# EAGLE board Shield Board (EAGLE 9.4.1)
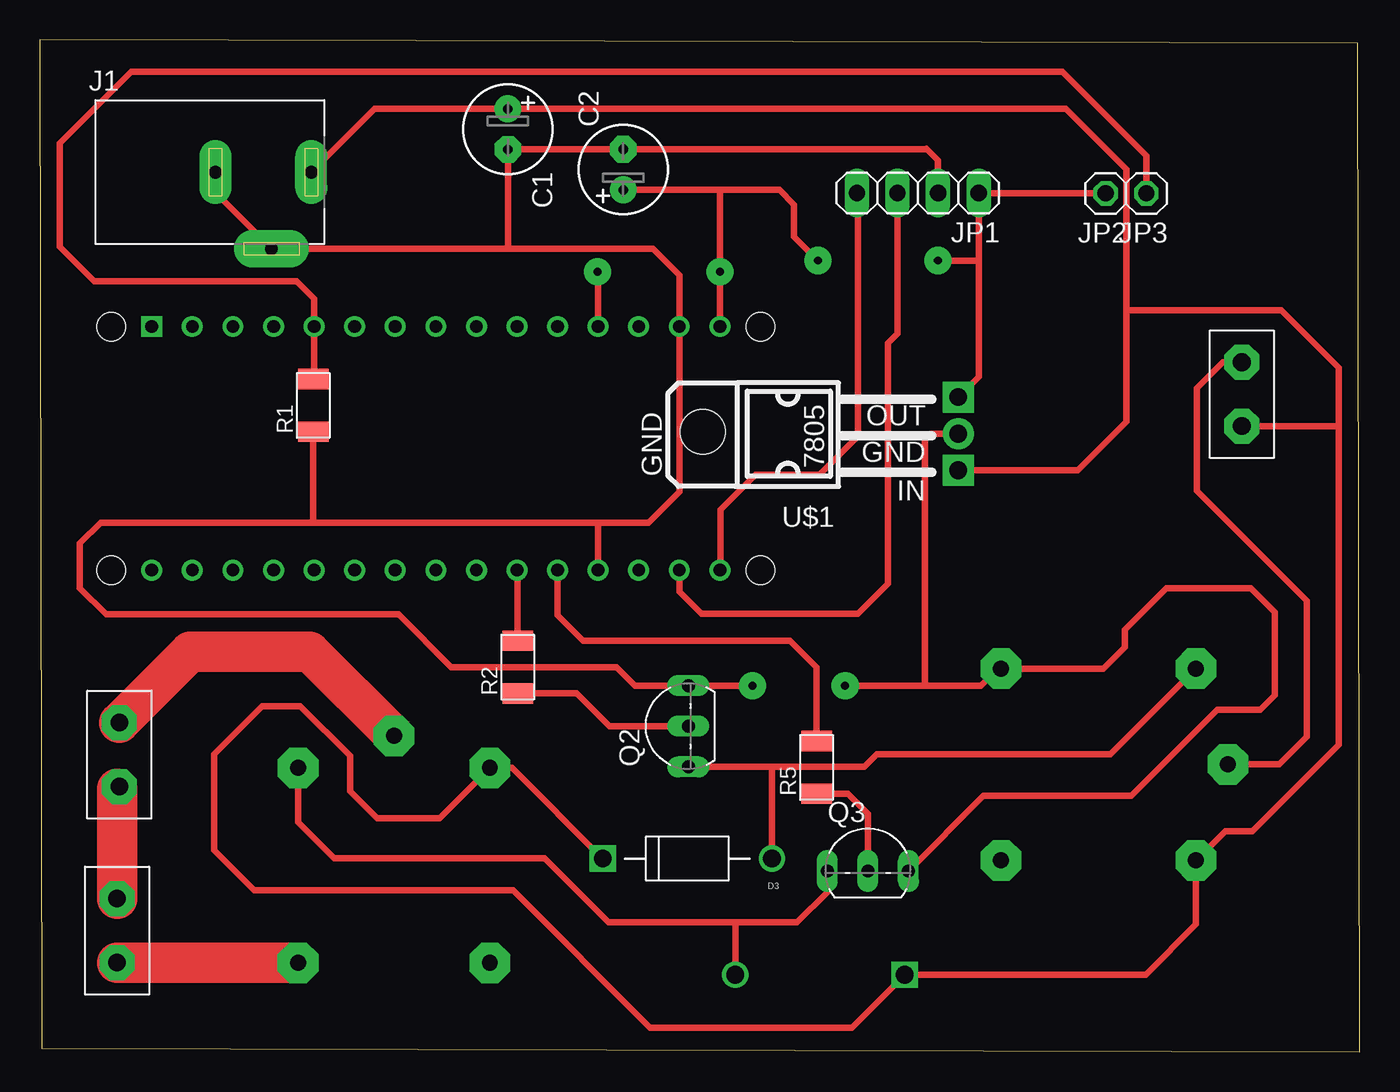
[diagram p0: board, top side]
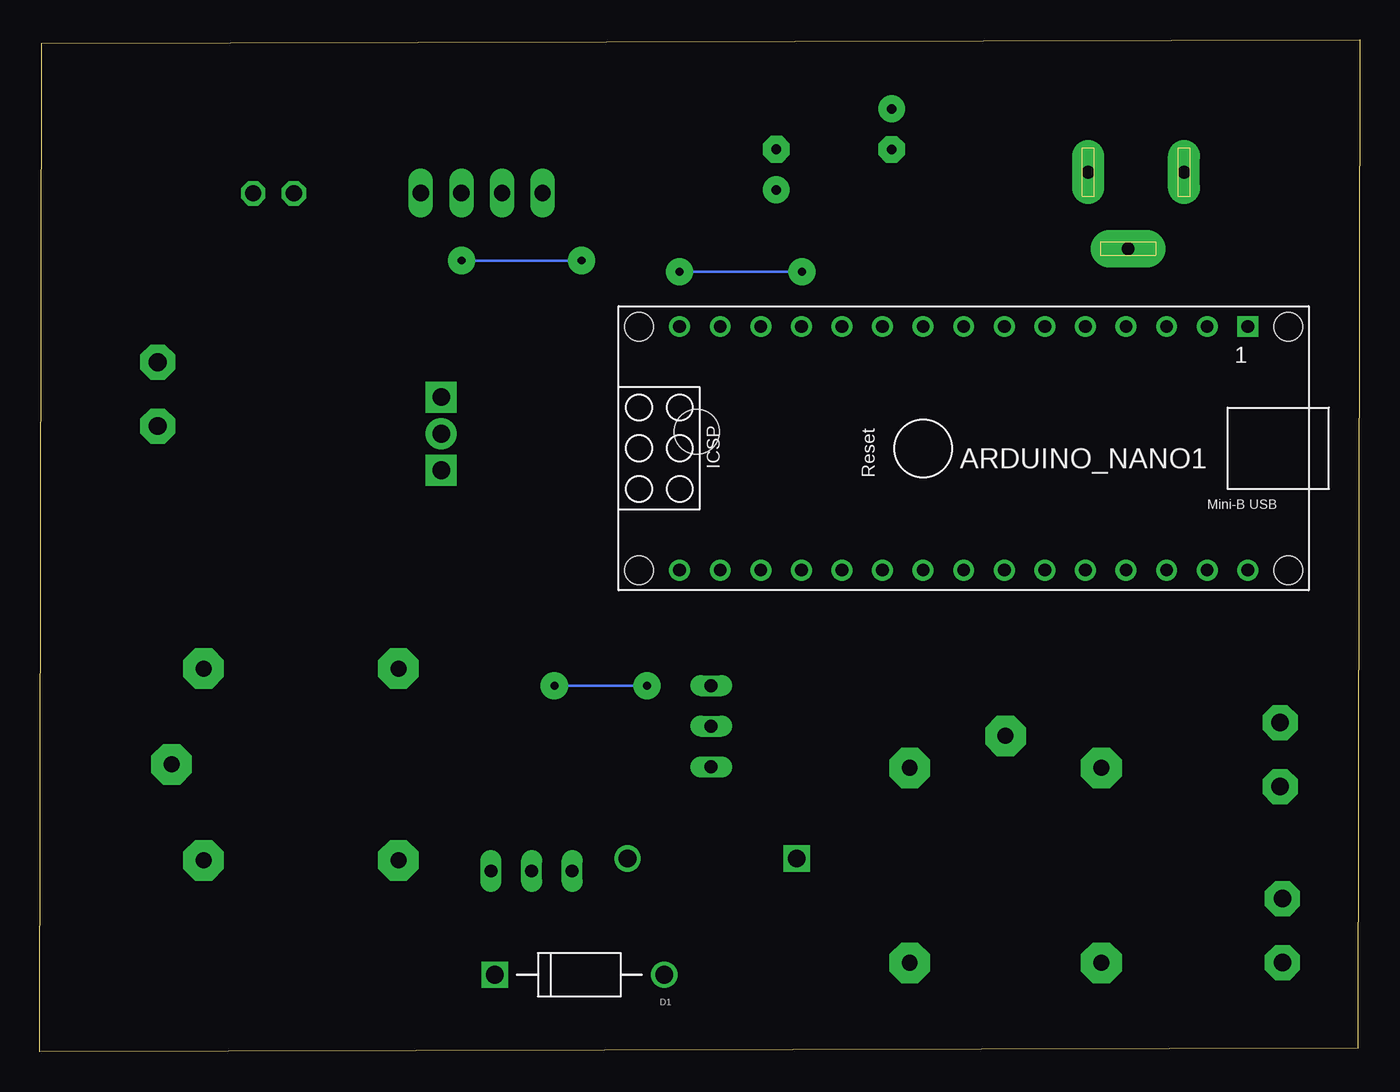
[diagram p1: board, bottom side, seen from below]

Size 82.6 x 63.3 mm. Coordinates in mm from the lower left corner, seen from the top.
Outline: 0.1,0.2 82.6,0 82.5,63.1 0,63.3 0.1,0.2
Copper layers (1*16): Top 0.035mm / dielectric 1.5mm / Bottom 0.035mm
Design rules "default": minimum track width 6mil, minimum drill 0.35mm, track to track 6mil, track to pad 6mil, pad to pad 6mil, via to via 6mil, smd to smd 6mil, copper to edge 40mil, drill to drill 6mil, minimum pad ring 10mil, minimum via ring 8mil, stop-mask expansion 4mil, vias tented up to drill 0mil, thermal gap 10mil

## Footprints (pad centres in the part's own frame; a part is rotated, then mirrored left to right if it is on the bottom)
ARDUINO_NANO = drill 0.8 square: 1 -20.32,-7.62 | drill 0.8: 2 -17.78,-7.62; 3 -15.24,-7.62; 4 -12.7,-7.62; 5 -10.16,-7.62; 6 -7.62,-7.62; 7 -5.08,-7.62; 8 -2.54,-7.62; 9 0,-7.62; 10 2.54,-7.62; 11 5.08,-7.62; 12 7.62,-7.62; 13 10.16,-7.62; 14 12.7,-7.62; 15 15.24,-7.62; 16 15.24,7.62; 17 12.7,7.62; 18 10.16,7.62; 19 7.62,7.62; 20 5.08,7.62; 21 2.54,7.62; 22 0,7.62; 23 -2.54,7.62; 24 -5.08,7.62; 25 -7.62,7.62; 26 -10.16,7.62; 27 -12.7,7.62; 28 -15.24,7.62; 29 -17.78,7.62; 30 -20.32,7.62 | hole 1.778: -22.86,-7.62; -22.86,7.62; 17.78,7.62; 17.78,-7.62
E2,5-6 = drill 0.6 pad 1.676: + -1.27,0 | drill 0.6 pad 1.676 octagon: - 1.27,0
DIOAD1060W80L520D270 = drill 1.1 pad 1.65: A 5.3,0 | drill 1.1 pad 1.65 square: C -5.3,0
NINIGI_DC-005 = drill 0.8 pad 2.35 long: 2 0,-4.8 | drill 0.8 pad 2 long: 3 -3.5,0; 4 2.5,0
1X04 = drill 1.016 long: 1 -3.81,0; 2 -1.27,0; 3 1.27,0; 4 3.81,0
1X01 = drill 1.016 octagon: 1 0,0
TO92-EBC = drill 0.813 long: B 0,-1.27; C -2.54,-1.27; E 2.54,-1.27
R1206FAB = smd 1.27 x 1.905: 1 -1.651,0; 2 1.651,0
L7805 = drill 1.1 pad 1.93: GND 0.127,-9.652 | drill 1.1 pad 1.93 square: IN -2.159,-9.652; OUT 2.413,-9.652 | hole 2.8: 0.254,6.35
RELAYSL = drill 1 pad 2.54 octagon: P$1 14.2,6; P$2 2,6; P$3 0,0; P$4 2,-6; P$5 14.2,-6
CNN = drill 1.1 pad 2.184 octagon: P$1 0,0; P$2 4,0

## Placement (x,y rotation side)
ARDUINO_NANO1  [ARDUINO_NANO]  27.32,37.75 180 bottom
C1  [E2,5-6]  29.29,57.72 270 top
C2  [E2,5-6]  36.51,55.19 90 top
D1  1N4007  [DIOAD1060W80L520D270]  48.83,4.81 0 bottom
D3  1N4007  [DIOAD1060W80L520D270]  40.52,12.08 0 top
J1  DC-005  [NINIGI_DC-005]  14.49,55.03 0 top
JP1  [1X04]  54.95,53.72 180 top
JP2  [1X01]  66.71,53.7 180 top
JP3  [1X01]  69.25,53.7 180 top
Q2  BC548  [TO92-EBC]  39.32,20.36 90 top
Q3  BC548  [TO92-EBC]  51.83,12.57 0 top
R1  1 K  [R1206FAB]  17.11,40.44 90 top
R2  1 K  [R1206FAB]  29.91,24.06 90 top
R5  1 K  [R1206FAB]  48.61,17.78 90 top
U$1  -L7805  [L7805]  47.83,38.54 90 top
U$3  RELAYSL  [RELAYSL]  74.36,17.97 180 top
U$5  RELAYSL  [RELAYSL]  22.16,19.75 270 top
U$6  CNN  [CNN]  4.83,9.57 270 top
U$7  CNN  [CNN]  4.97,16.58 90 top
U$8  CNN  [CNN]  75.23,43.14 270 top

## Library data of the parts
ARDUINO_NANO1 = ArduinoNanoV30
C1 C2 = Clean-Kong
D1 D3 = 1N4007; AVAILABILITY: Unavailable; DESCRIPTION: Diode, Standard Recovery, 1a, 1kv, Do-41, Full Reel; MF: Diodes; MP: 1N4007-T; PACKAGE: DO-41 Multicomp; PRICE: None
J1 = DC-005; AVAILABILITY: Unavailable; MF: Littelfuse Inc.; MP: DC-005; PACKAGE: 0603 Ninigi; PRICE: None
JP1-JP3 = pinhead
Q2 Q3 = transistor-npn
R1 R2 R5 = fab
U$1 = tango
U$3 U$5 = relay
U$6-U$8 = resistor-bourns

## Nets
5V: ARDUINO_NANO1.12 ARDUINO_NANO1.15 C2.+ JP1.1 JP2.1 U$1.OUT
GND: ARDUINO_NANO1.14 ARDUINO_NANO1.19 C1.- C2.- J1.2 J1.3 JP1.2 Q2.E Q3.E R1.1 U$1.GND U$3.P$5
N$3: D3.A Q2.C U$3.P$4
N$5: ARDUINO_NANO1.5 JP3.1 R1.2
N$6: Q2.B R2.1
N$8: ARDUINO_NANO1.21 R2.2
N$9: D1.A Q3.C U$5.P$4
N$11: Q3.B R5.1
N$12: ARDUINO_NANO1.20 R5.2
N$14: U$5.P$3 U$7.P$2
N$15: U$6.P$1 U$7.P$1
N$16: U$3.P$3 U$8.P$1
N$17: U$5.P$5 U$6.P$2
RX: ARDUINO_NANO1.16 JP1.4
TX: ARDUINO_NANO1.17 JP1.3
VCC: C1.+ D1.C D3.C J1.4 U$1.IN U$3.P$2 U$5.P$2 U$8.P$2

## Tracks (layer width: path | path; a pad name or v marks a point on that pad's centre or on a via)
5V  (via drill 0.5 pad 1.7)
  Top 0.152: 42.56,53.86 42.5,53.92 | JP1.1 58.8,53.72 58.82,53.7 | JP2.1 66.69,53.72 | 34.94,48.76 v34.9,48.8
  Top 0.406: v48.7,49.5 47.2,51 47.2,53 46.28,53.92 42.5,53.92 C2.+ | ARDUINO_NANO1.15 v42.56,48.8 42.56,53.86 | JP1.1 58.76,49.5 | 58.76,49.5 58.76,42.23 U$1.OUT | v56.2,49.5 58.76,49.5 | JP2.1 58.82,53.7 | ARDUINO_NANO1.12 34.94,48.76
  Bottom 0.152: v56.2,49.5 v48.7,49.5 | v34.9,48.8 v42.56,48.8 42.6,48.8
GND  (via drill 0.5 pad 1.7)
  Top 0.152: Q2.E | 36.48,56.45 C2.- | 15,50.23 J1.2 | 34.94,33.06 34.9,33.1 | 55.5,56.5 55.46,56.46 | 55.4,23 55.5,22.9 | 17.11,33.19 17.2,33.1 | 29.29,50.24 29.3,50.23 | J1.3 10.99,53.73
  Top 0.406: 36.48,56.45 C1.- 29.29,50.24 | ARDUINO_NANO1.19 34.94,33.06 | v44.6,22.9 Q2.E 37.24,22.9 36.09,24.05 25.75,24.05 22.45,27.35 4.15,27.35 2.5,29 2.5,31.8 3.8,33.1 17.2,33.1 34.9,33.1 38.1,33.1 40.02,35.02 ARDUINO_NANO1.14 40.02,48.58 38.37,50.23 29.3,50.23 J1.2 10.99,53.73 | v50.4,22.9 55.5,22.9 58.9,22.9 59.97,23.97 U$3.P$5 66.57,23.97 67.9,25.3 67.9,26.4 70.5,29 75.8,29 77.3,27.5 77.3,22.3 76.4,21.4 73.7,21.4 68.3,16 59.07,16 Q3.E | JP1.2 56.22,55.78 55.5,56.5 | 55.46,56.46 C2.- | U$1.GND 55.76,38.66 55.4,38.3 55.4,23 | R1.1 17.11,33.19
  Bottom 0.152: v44.6,22.9 v50.4,22.9
N$3
  Top 0.152: 51.68,17.82 51.6,17.82
  Top 0.406: Q2.C 45.82,17.82 | 45.82,17.82 51.6,17.82 52.38,18.6 66.99,18.6 U$3.P$4 | D3.A 45.82,17.82
N$5
  Top 0.152: 17.16,42.14 R1.2
  Top 0.406: JP3.1 69.25,56.05 64,61.3 5.7,61.3 1.25,56.85 1.25,50.35 3.4,48.2 16.06,48.2 17.16,47.1 ARDUINO_NANO1.5 17.16,42.14
N$6
  Top 0.406: R2.1 33.59,22.41 35.64,20.36 Q2.B
N$8
  Top 0.406: ARDUINO_NANO1.21 29.91,30.08 R2.2
N$9
  Top 0.406: U$5.P$4 16.16,14.34 18.4,12.1 31.6,12.1 35.6,8.1 43.53,8.1 | D1.A 43.53,8.1 | Q3.C 49.29,9.98 47.4,8.1 43.53,8.1
N$11
  Top 0.406: R5.1 50.57,16.13 51.83,14.88 Q3.B
N$12
  Top 0.406: R5.2 48.61,24.04 46.95,25.7 34,25.7 32.4,27.3 ARDUINO_NANO1.20
N$14
  Top 2.54: U$7.P$2 9.41,25.02 16.89,25.02 U$5.P$3
N$15
  Top 0.152: 4.83,16.44 U$7.P$1
  Top 2.54: U$6.P$1 4.83,16.44
N$16
  Top 0.406: U$3.P$3 77.57,17.97 79.3,19.7 79.3,28.2 72.4,35.1 72.4,41.5 74.03,43.14 U$8.P$1
N$17
  Top 0.152: 16.14,5.57 U$5.P$5
  Top 2.54: U$6.P$2 16.14,5.57
RX
  Top 0.152: ARDUINO_NANO1.16 42.6,30.17 | 51.2,53.66 JP1.4
  Top 0.406: 42.6,30.17 42.6,33.9 44.8,36.1 48.8,36.1 51.2,38.5 51.2,53.66
TX
  Top 0.406: JP1.3 53.68,44.92 53.08,44.32 53.08,29.28 51.2,27.4 41.4,27.4 40.02,28.78 ARDUINO_NANO1.17
VCC
  Top 0.152: 81.27,39.14 81.3,39.1 | 29.2,58.9 C1.+
  Top 0.406: D3.C 29.55,17.75 U$5.P$2 25.01,14.6 21.1,14.6 19.4,16.3 19.4,18.5 16.3,21.6 13.9,21.6 10.9,18.6 10.9,12.6 13.4,10.1 29.6,10.1 38.2,1.5 50.82,1.5 D1.C 69.21,4.81 72.36,7.96 U$3.P$2 74.19,13.8 75.9,13.8 81.3,19.2 81.3,39.1 81.3,42.8 77.7,46.4 68,46.4 | U$8.P$2 81.27,39.14 | J1.4 20.95,58.99 C1.+ 64.23,58.99 68,55.22 68,46.4 | 68,46.4 68,39.4 64.98,36.38 U$1.IN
